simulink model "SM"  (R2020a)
settings: Solver=VariableStepAuto  StartTime=0.0  StopTime=10  RelTol=1e-3
InitFcn:
  | initParams
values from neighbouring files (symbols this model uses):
  a = 10    [initParams.m]
  b = 1    [initParams.m]
  K = 10    [initParams.m]
  lambda = 1    [initParams.m]
  x0 = [0.2;0.1]    [initParams.m]

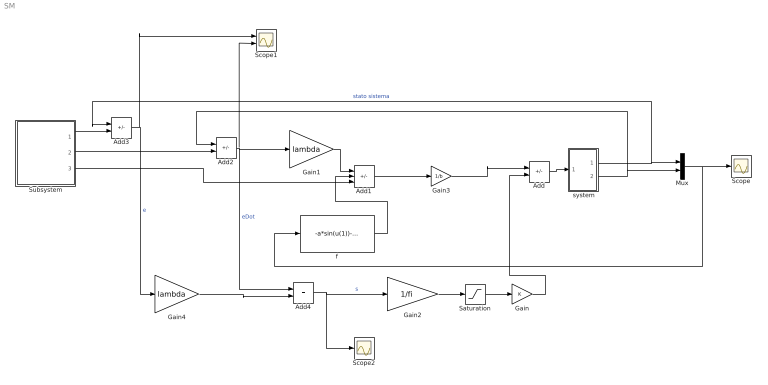
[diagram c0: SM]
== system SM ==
  " system" : Subsystem
  Add : Sum  Inputs=+-
  Add1 : Sum  Inputs=--+
  Add2 : Sum  Inputs=+-
  Add3 : Sum  Inputs=+-
  Add4 : Sum
  Gain : Gain  Gain=K
  Gain1 : Gain  Gain=lambda
  Gain2 : Gain  Gain=1/fi
  Gain3 : Gain  Gain=1/b
  Gain4 : Gain  Gain=lambda
  Mux : Mux  Inputs=2
  Saturation : Saturate  UpperLimit=1  LowerLimit=-1
  Scope : Scope
  Scope1 : Scope  NumInputPorts=2
  Scope2 : Scope
  Subsystem : Subsystem
  f : Fcn  Expr=-a*sin(u(1))-u(2)
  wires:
  " system"/1(x1) -> Add3/1, Mux/1  "stato sistema"
  " system"/2(x2) -> Add2/1, Mux/2
  Mux/1 -> f/1, Scope/1
  Gain2/1 -> Saturation/1
  Add/1 -> " system"/1(u)
  Add1/1 -> Gain3/1
  Subsystem/3(xDDot_d) -> Add1/3
  Gain3/1 -> Add/1
  f/1 -> Add1/2
  Gain1/1 -> Add1/1
  Subsystem/2(xDot_d) -> Add2/2
  Add2/1 -> Scope1/2, Add4/1, Gain1/1  "eDot"
  Subsystem/1(x_d) -> Add3/2
  Add3/1 -> Scope1/1, Gain4/1  "e"
  Gain4/1 -> Add4/2
  Add4/1 -> Scope2/1, Gain2/1  "s"
  Saturation/1 -> Gain/1
  Gain/1 -> Add/2

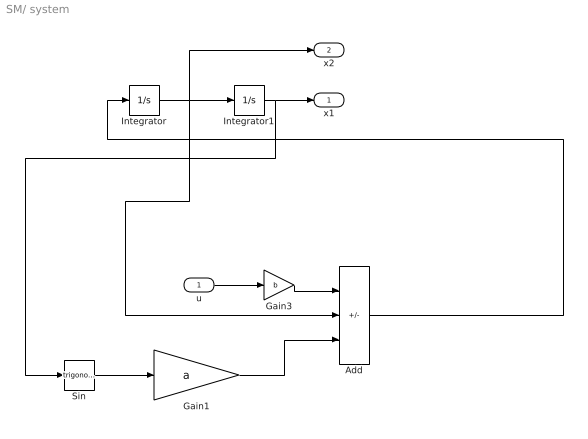
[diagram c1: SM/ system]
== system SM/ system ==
  u : Inport
  Add : Sum  Inputs=+--
  Gain1 : Gain  Gain=a
  Gain3 : Gain  Gain=b
  Integrator : Integrator  InitialCondition=x0(2)
  Integrator1 : Integrator  InitialCondition=x0(1)
  Sin : Trigonometry
  x1 : Outport
  x2 : Outport  Port=2
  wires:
  Add/1 -> Integrator/1
  Gain3/1 -> Add/1
  Gain1/1 -> Add/3
  Sin/1 -> Gain1/1
  u/1 -> Gain3/1
  Integrator1/1 -> Sin/1, x1/1
  Integrator/1 -> Add/2, x2/1, Integrator1/1

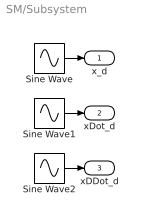
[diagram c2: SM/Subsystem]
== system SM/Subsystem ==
  Sine Wave : Sin  SampleTime=0
  Sine Wave1 : Sin  Phase=pi/2  SampleTime=0
  Sine Wave2 : Sin  Amplitude=-1  SampleTime=0
  x_d : Outport
  xDot_d : Outport  Port=2
  xDDot_d : Outport  Port=3
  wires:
  Sine Wave/1 -> x_d/1
  Sine Wave2/1 -> xDDot_d/1
  Sine Wave1/1 -> xDot_d/1
